| IBIS file stm32l0_31_41_wlcsp25.ibs
| Created by s2ibis version 1.1 (customized version)
| North Carolina State University, ERL, 2006
[IBIS ver] 4.2
[File name] stm32l0_31_41_wlcsp25.ibs
[File Rev] 1.0
[Date]  14-03-2016
[Source] Data Created at STMicroelectronics
[Notes]  File originated from ELDO simulations.
[Disclaimer]  This information is for modeling purpose only and is
   not guaranted. The information is subject to change without
   notice.
[Copyright] Copyright 2016 STMicroelectronics Inc.
|   Component stm32l0_31_41_wlcsp25
[Component] stm32l0_31_41_wlcsp25
[Manufacturer] STMicroelectronics
[Package]
| variable   typ   min   max
R_pkg   0.0   0.0   0.0
L_pkg   0.0H   0.0H   0.0H
C_pkg   0.0F   0.0F   0.0F
[Pin]  signal_name   model_name   R_pin   L_pin   C_pin
B5 PC14-OSC32_IN io8p_wsudq_ls_ft_v33
C5 PC15-OSC32_OUT io8p_sudq_ls_tc_esdft
D5 NRST ioreset_ft_v33
E1 VSSA GND
C4 VDDA POWER
E5 PA0 io8p_wsudq_ls_ft_v33
B4 PA1 io8p_wsudq_lcd4_ls_ft
D4 PA2 io8p_wsudq_ls_ft_v33
E4 PA3 io8p_wsudq_lcd4_ls_ft
B3 PA4 io8p_wsudq_i2cin_ls_ft
D3 PA5 io8p_wsudq_i2cin_ls_ft
E3 PA6 io8p_wsudq_lcd4_ls_ft
C3 PA7 io8p_wsudq_lcd4_ls_ft
E2 PB0 io8p_wsudq_lcd4_ls_ft
D2 PB1 io8p_wsudq_lcd4_ls_ft
C1 PA8 io8p_sudq_ls_ft
B1 PA9 io8p_sudq_lcd4_i2cin_ls_ft
C2 PA10 io8p_sudq_lcd4_i2cin_ls_ft
A1 PA13 io8p_sudq_ls_ft
D1 VDD POWER
A2 PA14 io8p_sudq_ls_ft
B2 PB3 io8p_sudq_ls_ft
A3 PB6 io8p_sudq_lcd4_i2cin_ls_ft
A4 PB7 io8p_wsudq_i2cin_ls_ft
A5 BOOT0 vpp_test_hv
[Model Selector] io8p_sudq_ls_ft
io8p00_sudq_ls_ft_pd_lv  "SPEED00 1P8V, PD=40kOhm"
io8p00_sudq_ls_ft_pu_lv  "SPEED00 1P8V, PU=40kOhm"
io8p00_sudq_ls_ft_lv  "SPEED00 1P8V"
io8p01_sudq_ls_ft_pd_lv  "SPEED01 1P8V, PD=40kOhm"
io8p01_sudq_ls_ft_pu_lv  "SPEED01 1P8V, PU=40kOhm"
io8p01_sudq_ls_ft_lv  "SPEED01 1P8V"
io8p10_sudq_ls_ft_pd_lv  "SPEED10 1P8V, PD=40kOhm"
io8p10_sudq_ls_ft_pu_lv  "SPEED10 1P8V, PU=40kOhm"
io8p10_sudq_ls_ft_lv  "SPEED10 1P8V"
io8p11_sudq_ls_ft_pd_lv  "SPEED11 1P8V, PD=40kOhm"
io8p11_sudq_ls_ft_pu_lv  "SPEED11 1P8V, PU=40kOhm"
io8p11_sudq_ls_ft_lv  "SPEED11 1P8V"
io8p00_sudq_ls_ft_pd  "SPEED00, PD=40kOhm"
io8p00_sudq_ls_ft_pu  "SPEED00, PU=40kOhm"
io8p00_sudq_ls_ft  "SPEED00"
io8p01_sudq_ls_ft_pd  "SPEED01, PD=40kOhm"
io8p01_sudq_ls_ft_pu  "SPEED01, PU=40kOhm"
io8p01_sudq_ls_ft  "SPEED01"
io8p10_sudq_ls_ft_pd  "SPEED10, PD=40kOhm"
io8p10_sudq_ls_ft_pu  "SPEED10, PU=40kOhm"
io8p10_sudq_ls_ft  "SPEED10"
io8p11_sudq_ls_ft_pd  "SPEED11, PD=40kOhm"
io8p11_sudq_ls_ft_pu  "SPEED11, PU=40kOhm"
io8p11_sudq_ls_ft  "SPEED11"
[Model Selector] io8p_sudq_ls_tc_esdft
io8p00_sudq_ls_tc_esdft_pd_lv  "SPEED00 1P8V, PD=40kOhm"
io8p00_sudq_ls_tc_esdft_pu_lv  "SPEED00 1P8V, PU=40kOhm"
io8p00_sudq_ls_tc_esdft_lv  "SPEED00 1P8V"
io8p01_sudq_ls_tc_esdft_pd_lv  "SPEED01 1P8V, PD=40kOhm"
io8p01_sudq_ls_tc_esdft_pu_lv  "SPEED01 1P8V, PU=40kOhm"
io8p01_sudq_ls_tc_esdft_lv  "SPEED01 1P8V"
io8p10_sudq_ls_tc_esdft_pd_lv  "SPEED10 1P8V, PD=40kOhm"
io8p10_sudq_ls_tc_esdft_pu_lv  "SPEED10 1P8V, PU=40kOhm"
io8p10_sudq_ls_tc_esdft_lv  "SPEED10 1P8V"
io8p11_sudq_ls_tc_esdft_pd_lv  "SPEED11 1P8V, PD=40kOhm"
io8p11_sudq_ls_tc_esdft_pu_lv  "SPEED11 1P8V, PU=40kOhm"
io8p11_sudq_ls_tc_esdft_lv  "SPEED11 1P8V"
io8p00_sudq_ls_tc_esdft_pd  "SPEED00, PD=40kOhm"
io8p00_sudq_ls_tc_esdft_pu  "SPEED00, PU=40kOhm"
io8p00_sudq_ls_tc_esdft  "SPEED00"
io8p01_sudq_ls_tc_esdft_pd  "SPEED01, PD=40kOhm"
io8p01_sudq_ls_tc_esdft_pu  "SPEED01, PU=40kOhm"
io8p01_sudq_ls_tc_esdft  "SPEED01"
io8p10_sudq_ls_tc_esdft_pd  "SPEED10, PD=40kOhm"
io8p10_sudq_ls_tc_esdft_pu  "SPEED10, PU=40kOhm"
io8p10_sudq_ls_tc_esdft  "SPEED10"
io8p11_sudq_ls_tc_esdft_pd  "SPEED11, PD=40kOhm"
io8p11_sudq_ls_tc_esdft_pu  "SPEED11, PU=40kOhm"
io8p11_sudq_ls_tc_esdft  "SPEED11"
[Model Selector] io8p_wsudq_i2cin_ls_ft
io8p00_wsudq_i2cin_ls_ft_pd_lv  "SPEED00 1P8V, PD=40kOhm"
io8p00_wsudq_i2cin_ls_ft_pu_lv  "SPEED00 1P8V, PU=40kOhm"
io8p00_wsudq_i2cin_ls_ft_lv  "SPEED00 1P8V"
io8p01_wsudq_i2cin_ls_ft_pd_lv  "SPEED01 1P8V, PD=40kOhm"
io8p01_wsudq_i2cin_ls_ft_pu_lv  "SPEED01 1P8V, PU=40kOhm"
io8p01_wsudq_i2cin_ls_ft_lv  "SPEED01 1P8V"
io8p10_wsudq_i2cin_ls_ft_pd_lv  "SPEED10 1P8V, PD=40kOhm"
io8p10_wsudq_i2cin_ls_ft_pu_lv  "SPEED10 1P8V, PU=40kOhm"
io8p10_wsudq_i2cin_ls_ft_lv  "SPEED10 1P8V"
io8p11_wsudq_i2cin_ls_ft_pd_lv  "SPEED11 1P8V, PD=40kOhm"
io8p11_wsudq_i2cin_ls_ft_pu_lv  "SPEED11 1P8V, PU=40kOhm"
io8p11_wsudq_i2cin_ls_ft_lv  "SPEED11 1P8V"
io8p00_wsudq_i2cin_ls_ft_pd  "SPEED00, PD=40kOhm"
io8p00_wsudq_i2cin_ls_ft_pu  "SPEED00, PU=40kOhm"
io8p00_wsudq_i2cin_ls_ft  "SPEED00"
io8p01_wsudq_i2cin_ls_ft_pd  "SPEED01, PD=40kOhm"
io8p01_wsudq_i2cin_ls_ft_pu  "SPEED01, PU=40kOhm"
io8p01_wsudq_i2cin_ls_ft  "SPEED01"
io8p10_wsudq_i2cin_ls_ft_pd  "SPEED10, PD=40kOhm"
io8p10_wsudq_i2cin_ls_ft_pu  "SPEED10, PU=40kOhm"
io8p10_wsudq_i2cin_ls_ft  "SPEED10"
io8p11_wsudq_i2cin_ls_ft_pd  "SPEED11, PD=40kOhm"
io8p11_wsudq_i2cin_ls_ft_pu  "SPEED11, PU=40kOhm"
io8p11_wsudq_i2cin_ls_ft  "SPEED11"
[Model Selector] io8p_wsudq_lcd4_ls_ft
io8p00_wsudq_lcd4_ls_ft_pd_lv  "SPEED00 1P8V, PD=40kOhm"
io8p00_wsudq_lcd4_ls_ft_pu_lv  "SPEED00 1P8V, PU=40kOhm"
io8p00_wsudq_lcd4_ls_ft_lv  "SPEED00 1P8V"
io8p01_wsudq_lcd4_ls_ft_pd_lv  "SPEED01 1P8V, PD=40kOhm"
io8p01_wsudq_lcd4_ls_ft_pu_lv  "SPEED01 1P8V, PU=40kOhm"
io8p01_wsudq_lcd4_ls_ft_lv  "SPEED01 1P8V"
io8p10_wsudq_lcd4_ls_ft_pd_lv  "SPEED10 1P8V, PD=40kOhm"
io8p10_wsudq_lcd4_ls_ft_pu_lv  "SPEED10 1P8V, PU=40kOhm"
io8p10_wsudq_lcd4_ls_ft_lv  "SPEED10 1P8V"
io8p11_wsudq_lcd4_ls_ft_pd_lv  "SPEED11 1P8V, PD=40kOhm"
io8p11_wsudq_lcd4_ls_ft_pu_lv  "SPEED11 1P8V, PU=40kOhm"
io8p11_wsudq_lcd4_ls_ft_lv  "SPEED11 1P8V"
io8p00_wsudq_lcd4_ls_ft_pd  "SPEED00, PD=40kOhm"
io8p00_wsudq_lcd4_ls_ft_pu  "SPEED00, PU=40kOhm"
io8p00_wsudq_lcd4_ls_ft  "SPEED00"
io8p01_wsudq_lcd4_ls_ft_pd  "SPEED01, PD=40kOhm"
io8p01_wsudq_lcd4_ls_ft_pu  "SPEED01, PU=40kOhm"
io8p01_wsudq_lcd4_ls_ft  "SPEED01"
io8p10_wsudq_lcd4_ls_ft_pd  "SPEED10, PD=40kOhm"
io8p10_wsudq_lcd4_ls_ft_pu  "SPEED10, PU=40kOhm"
io8p10_wsudq_lcd4_ls_ft  "SPEED10"
io8p11_wsudq_lcd4_ls_ft_pd  "SPEED11, PD=40kOhm"
io8p11_wsudq_lcd4_ls_ft_pu  "SPEED11, PU=40kOhm"
io8p11_wsudq_lcd4_ls_ft  "SPEED11"
[Model Selector] io8p_wsudq_ls_ft_v33
io8p00_wsudq_ls_ft_v33_pd_lv  "SPEED00 1P8V, PD=40kOhm"
io8p00_wsudq_ls_ft_v33_pu_lv  "SPEED00 1P8V, PU=40kOhm"
io8p00_wsudq_ls_ft_v33_lv  "SPEED00 1P8V"
io8p01_wsudq_ls_ft_v33_pd_lv  "SPEED01 1P8V, PD=40kOhm"
io8p01_wsudq_ls_ft_v33_pu_lv  "SPEED01 1P8V, PU=40kOhm"
io8p01_wsudq_ls_ft_v33_lv  "SPEED01 1P8V"
io8p10_wsudq_ls_ft_v33_pd_lv  "SPEED10 1P8V, PD=40kOhm"
io8p10_wsudq_ls_ft_v33_pu_lv  "SPEED10 1P8V, PU=40kOhm"
io8p10_wsudq_ls_ft_v33_lv  "SPEED10 1P8V"
io8p11_wsudq_ls_ft_v33_pd_lv  "SPEED11 1P8V, PD=40kOhm"
io8p11_wsudq_ls_ft_v33_pu_lv  "SPEED11 1P8V, PU=40kOhm"
io8p11_wsudq_ls_ft_v33_lv  "SPEED11 1P8V"
io8p00_wsudq_ls_ft_v33_pd  "SPEED00, PD=40kOhm"
io8p00_wsudq_ls_ft_v33_pu  "SPEED00, PU=40kOhm"
io8p00_wsudq_ls_ft_v33  "SPEED00"
io8p01_wsudq_ls_ft_v33_pd  "SPEED01, PD=40kOhm"
io8p01_wsudq_ls_ft_v33_pu  "SPEED01, PU=40kOhm"
io8p01_wsudq_ls_ft_v33  "SPEED01"
io8p10_wsudq_ls_ft_v33_pd  "SPEED10, PD=40kOhm"
io8p10_wsudq_ls_ft_v33_pu  "SPEED10, PU=40kOhm"
io8p10_wsudq_ls_ft_v33  "SPEED10"
io8p11_wsudq_ls_ft_v33_pd  "SPEED11, PD=40kOhm"
io8p11_wsudq_ls_ft_v33_pu  "SPEED11, PU=40kOhm"
io8p11_wsudq_ls_ft_v33  "SPEED11"
[Model Selector] vpp_test_hv
vpp_test_hv_2p4  "Input Buffer 1P65V"
vpp_test_hv_3p3  "Input Buffer"
[Model Selector] io8p_sudq_lcd4_i2cin_ls_ft
io8p00_sudq_lcd4_i2cin_ls_ft_pd_lv  "SPEED00 1P8V, PD=40kOhm"
io8p00_sudq_lcd4_i2cin_ls_ft_pu_lv  "SPEED00 1P8V, PU=40kOhm"
io8p00_sudq_lcd4_i2cin_ls_ft_lv  "SPEED00 1P8V"
io8p01_sudq_lcd4_i2cin_ls_ft_pd_lv  "SPEED01 1P8V, PD=40kOhm"
io8p01_sudq_lcd4_i2cin_ls_ft_pu_lv  "SPEED01 1P8V, PU=40kOhm"
io8p01_sudq_lcd4_i2cin_ls_ft_lv  "SPEED01 1P8V"
io8p10_sudq_lcd4_i2cin_ls_ft_pd_lv  "SPEED10 1P8V, PD=40kOhm"
io8p10_sudq_lcd4_i2cin_ls_ft_pu_lv  "SPEED10 1P8V, PU=40kOhm"
io8p10_sudq_lcd4_i2cin_ls_ft_lv  "SPEED10 1P8V"
io8p11_sudq_lcd4_i2cin_ls_ft_pd_lv  "SPEED11 1P8V, PD=40kOhm"
io8p11_sudq_lcd4_i2cin_ls_ft_pu_lv  "SPEED11 1P8V, PU=40kOhm"
io8p11_sudq_lcd4_i2cin_ls_ft_lv  "SPEED11 1P8V"
io8p00_sudq_lcd4_i2cin_ls_ft_pd  "SPEED00, PD=40kOhm"
io8p00_sudq_lcd4_i2cin_ls_ft_pu  "SPEED00, PU=40kOhm"
io8p00_sudq_lcd4_i2cin_ls_ft  "SPEED00"
io8p01_sudq_lcd4_i2cin_ls_ft_pd  "SPEED01, PD=40kOhm"
io8p01_sudq_lcd4_i2cin_ls_ft_pu  "SPEED01, PU=40kOhm"
io8p01_sudq_lcd4_i2cin_ls_ft  "SPEED01"
io8p10_sudq_lcd4_i2cin_ls_ft_pd  "SPEED10, PD=40kOhm"
io8p10_sudq_lcd4_i2cin_ls_ft_pu  "SPEED10, PU=40kOhm"
io8p10_sudq_lcd4_i2cin_ls_ft  "SPEED10"
io8p11_sudq_lcd4_i2cin_ls_ft_pd  "SPEED11, PD=40kOhm"
io8p11_sudq_lcd4_i2cin_ls_ft_pu  "SPEED11, PU=40kOhm"
io8p11_sudq_lcd4_i2cin_ls_ft  "SPEED11"
[Model Selector] ioreset_ft_v33
ioreset_ft_v33_pu_lv  "ioreset 1P8V + PU=40kOhm"
ioreset_ft_v33_nopu_lv  "ioreset 1P8V"
ioreset_ft_v33_pu  "ioreset + PU=40kOhm"
ioreset_ft_v33_nopu  "ioreset"
| Models and submodels in the file (150): io8p00_sudq_ls_ft_pd_lv (I/O), io8p00_sudq_ls_ft_pu_lv (I/O), io8p00_sudq_ls_ft_lv (I/O), io8p01_sudq_ls_ft_pd_lv (I/O), io8p01_sudq_ls_ft_pu_lv (I/O), io8p01_sudq_ls_ft_lv (I/O), io8p10_sudq_ls_ft_pd_lv (I/O), io8p10_sudq_ls_ft_pu_lv (I/O), io8p10_sudq_ls_ft_lv (I/O), io8p11_sudq_ls_ft_pd_lv (I/O), io8p11_sudq_ls_ft_pu_lv (I/O), io8p11_sudq_ls_ft_lv (I/O), io8p00_sudq_ls_ft_pd (I/O), io8p00_sudq_ls_ft_pu (I/O), io8p00_sudq_ls_ft (I/O), io8p01_sudq_ls_ft_pd (I/O), io8p01_sudq_ls_ft_pu (I/O), io8p01_sudq_ls_ft (I/O), io8p10_sudq_ls_ft_pd (I/O), io8p10_sudq_ls_ft_pu (I/O), io8p10_sudq_ls_ft (I/O), io8p11_sudq_ls_ft_pd (I/O), io8p11_sudq_ls_ft_pu (I/O), io8p11_sudq_ls_ft (I/O), io8p00_sudq_ls_tc_esdft_pd_lv (I/O), io8p00_sudq_ls_tc_esdft_pu_lv (I/O), io8p00_sudq_ls_tc_esdft_lv (I/O), io8p01_sudq_ls_tc_esdft_pd_lv (I/O), io8p01_sudq_ls_tc_esdft_pu_lv (I/O), io8p01_sudq_ls_tc_esdft_lv (I/O), io8p10_sudq_ls_tc_esdft_pd_lv (I/O), io8p10_sudq_ls_tc_esdft_pu_lv (I/O), io8p10_sudq_ls_tc_esdft_lv (I/O), io8p11_sudq_ls_tc_esdft_pd_lv (I/O), io8p11_sudq_ls_tc_esdft_pu_lv (I/O), io8p11_sudq_ls_tc_esdft_lv (I/O), io8p00_sudq_ls_tc_esdft_pd (I/O), io8p00_sudq_ls_tc_esdft_pu (I/O), io8p00_sudq_ls_tc_esdft (I/O), io8p01_sudq_ls_tc_esdft_pd (I/O), io8p01_sudq_ls_tc_esdft_pu (I/O), io8p01_sudq_ls_tc_esdft (I/O), io8p10_sudq_ls_tc_esdft_pd (I/O), io8p10_sudq_ls_tc_esdft_pu (I/O), io8p10_sudq_ls_tc_esdft (I/O), io8p11_sudq_ls_tc_esdft_pd (I/O), io8p11_sudq_ls_tc_esdft_pu (I/O), io8p11_sudq_ls_tc_esdft (I/O), io8p00_wsudq_i2cin_ls_ft_pd_lv (I/O), io8p00_wsudq_i2cin_ls_ft_pu_lv (I/O), io8p00_wsudq_i2cin_ls_ft_lv (I/O), io8p01_wsudq_i2cin_ls_ft_pd_lv (I/O), io8p01_wsudq_i2cin_ls_ft_pu_lv (I/O), io8p01_wsudq_i2cin_ls_ft_lv (I/O), io8p10_wsudq_i2cin_ls_ft_pd_lv (I/O), io8p10_wsudq_i2cin_ls_ft_pu_lv (I/O), io8p10_wsudq_i2cin_ls_ft_lv (I/O), io8p11_wsudq_i2cin_ls_ft_pd_lv (I/O), io8p11_wsudq_i2cin_ls_ft_pu_lv (I/O), io8p11_wsudq_i2cin_ls_ft_lv (I/O), io8p00_wsudq_i2cin_ls_ft_pd (I/O), io8p00_wsudq_i2cin_ls_ft_pu (I/O), io8p00_wsudq_i2cin_ls_ft (I/O), io8p01_wsudq_i2cin_ls_ft_pd (I/O), io8p01_wsudq_i2cin_ls_ft_pu (I/O), io8p01_wsudq_i2cin_ls_ft (I/O), io8p10_wsudq_i2cin_ls_ft_pd (I/O), io8p10_wsudq_i2cin_ls_ft_pu (I/O), io8p10_wsudq_i2cin_ls_ft (I/O), io8p11_wsudq_i2cin_ls_ft_pd (I/O), io8p11_wsudq_i2cin_ls_ft_pu (I/O), io8p11_wsudq_i2cin_ls_ft (I/O), io8p00_wsudq_lcd4_ls_ft_pd_lv (I/O), io8p00_wsudq_lcd4_ls_ft_pu_lv (I/O), io8p00_wsudq_lcd4_ls_ft_lv (I/O), io8p01_wsudq_lcd4_ls_ft_pd_lv (I/O), io8p01_wsudq_lcd4_ls_ft_pu_lv (I/O), io8p01_wsudq_lcd4_ls_ft_lv (I/O), io8p10_wsudq_lcd4_ls_ft_pd_lv (I/O), io8p10_wsudq_lcd4_ls_ft_pu_lv (I/O)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
